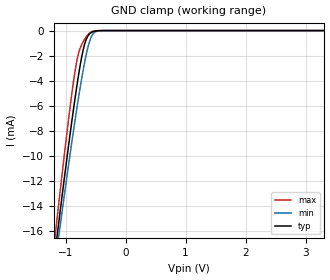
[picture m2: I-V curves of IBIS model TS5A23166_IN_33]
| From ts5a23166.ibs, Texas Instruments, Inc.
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[Model]   TS5A23166_IN_33
Model_type  Input
Vinl=0.8
Vinh=2
| variable   typ   min   max
C_comp   1.61pF   1.30pF   2.02pF
[Temperature Range]   40   100   -40
| Ambient temperature   25   85   -40
[Voltage range]   3.3   3   3.6
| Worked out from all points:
|   GND clamp passes 1 mA (typ) near -0.68 V on its own axis
[GND Clamp]
| TS5A23166_IN_33
|   Voltage   I(typ)   I(min)   I(max)
-3.3V     -108.5mA   -102.4mA   -115.8mA
-1.165V   -17.38mA   -18.31mA   -16.07mA
-1.14V    -16.4mA    -17.41mA   -14.99mA
-1.11V    -15.23mA   -16.34mA   -13.7mA
-1.085V   -14.27mA   -15.45mA   -12.64mA
-920mV    -8.126mA   -9.736mA   -5.957mA
-820mV    -4.705mA   -6.482mA   -2.626mA
-765mV    -3.026mA   -4.805mA   -1.531mA
-690mV    -1.227mA   -2.737mA   -750.6uA
-570mV    -154.4uA   -498.4uA   -105.7uA
-375mV    -1.348uA   -3.159uA   -200.4nA
3.3V      59.53pA    137.9pA    39.69pA
